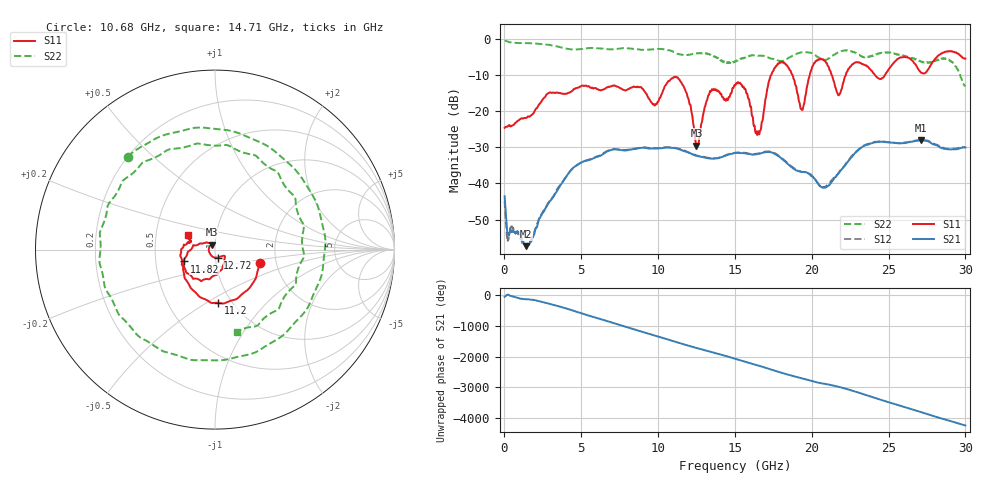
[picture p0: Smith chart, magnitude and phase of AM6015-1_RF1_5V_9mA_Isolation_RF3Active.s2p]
!Agilent Technologies,E8364B,MY43040894,A.07.50.67
!Agilent E8364B: A.07.50.67
!Date: Monday, August 13, 2018 07:02:25
!Correction: S11(Full 2 Port(1,2))
!S21(Full 2 Port(1,2))
!S12(Full 2 Port(1,2))
!S22(Full 2 Port(1,2))
!S2P File: Measurements: S11, S21, S12, S22:
# Hz S  dB  R 50
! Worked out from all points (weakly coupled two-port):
!   1601 points, 10 MHz to 30 GHz, reference 50 ohm
!   highest |S21| = -28.02 dB at 27.09 GHz (marker M1); lowest = -57.4 dB at 1.416 GHz (marker M2)
!   lowest |S11| = -29.5 dB at 12.49 GHz (marker M3), VSWR 1.07, Z = 48 + j2.65 ohm
!   |S11| at or under -10 dB: start of sweep to 17.33 GHz; 18.76 GHz to 19.87 GHz (1.108 GHz wide, 5.74 % of centre); 21.31 GHz to 22.21 GHz (893.3 MHz wide, 4.11 % of centre)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
!   |S22| runs from -12.9 to -0.3 dB; largest |S21 - S12| = 0.012
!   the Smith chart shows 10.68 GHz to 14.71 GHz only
!   S11 on the Smith chart (normalised r, x): 10.68 GHz: 1.65, -0.27; 11.2 GHz: 0.87, -0.56; 11.82 GHz: 0.70, -0.10; 12.72 GHz: 1.03, -0.09; 14.71 GHz: 0.73, +0.13
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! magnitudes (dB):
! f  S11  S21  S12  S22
! 10 MHz  -24.6  -43.6  -44.9  -0.3
! 1.416 GHz  -21.8  -57.4  -57.3  -1.0
! 5.015 GHz  -12.9  -34.2  -34.1  -2.7
! 10.02 GHz  -17.3  -30.3  -30.2  -2.7
! 10.68 GHz  -11.6  -30.0  -29.9  -3.0
! 11.2 GHz  -10.5  -30.3  -30.2  -3.9
! 11.82 GHz  -14.7  -31.2  -31.0  -4.4
! 12.49 GHz  -29.5  -32.3  -32.2  -3.9
! 12.72 GHz  -26.6  -32.5  -32.4  -3.8
! 13.39 GHz  -14.3  -33.1  -33.0  -4.3
! 14.71 GHz  -15.2  -31.8  -31.7  -6.5
! 15.01 GHz  -12.7  -31.6  -31.5  -6.1
! 16.49 GHz  -26.2  -31.8  -31.7  -4.5
! 17.69 GHz  -7.3  -32.0  -31.8  -5.7
! 19.35 GHz  -19.5  -36.8  -36.8  -3.6
! 20.01 GHz  -7.9  -38.0  -37.8  -3.8
! 20.83 GHz  -5.9  -41.1  -40.9  -5.7
! 21.75 GHz  -15.5  -37.1  -37.1  -3.6
! 22.76 GHz  -6.6  -31.8  -31.7  -3.5
! 25.01 GHz  -8.2  -28.6  -28.6  -3.6
! 27.09 GHz  -9.2  -28.0  -27.8  -6.2
! 30 GHz  -5.3  -30.0  -29.9  -12.7
